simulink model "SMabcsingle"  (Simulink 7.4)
settings: Solver=ode45  StartTime=0.0  StopTime=16  MaxStep=2e-4
InitFcn:
  | smparamsingle
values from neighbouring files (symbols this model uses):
  Bm = 0.10    (= 0.1)    [IMabc2.m]    (also in imabcparam.m = 0.01; IMabcrun0.m = 0.01; IMabcrun1.m = 0.001; IMcur0.m = 1e-06)
  D = str2num(get(h,'string'))    [acttrcalc1.m]
  J = 0.02    [imabcparam.m]    (also in IMabcrun0.m; IMabcrun1.m; imdefSIvec1.m = 0.03)
  Lm = eval(get(hLm,'String'))    [im3d.m]    (also in IMabc2.m = 4.5; imabcparam.m = 0.0847; IMabcrun0.m = 0.0847; IMabcrun1.m = 0.0847)
  Lr = Lrl+Lm    (= 4.6)    [IMabc2.m]    (also in IMabcf0.m = Lrl+Lm1; IMabcf1.m = Lrl+Lm1; imabcparam.m = 0.0589666666667; IMcur0.m)
  Ls = Lsl+Lm    (= 4.6)    [IMabc2.m]    (also in IMabcf0.m = Lsl+Lm1; IMabcf1.m = Lsl+Lm1; imabcparam.m = 0.0589666666667; IMcur0.m)
  nsync = 120*freq0/p    (= 1800)    [imabcparam.m]
  p = cos(beta-alpha)    [abcRwdg.m]    (also in alternator.m = 0:pi/20:2*pi; altwdgs.m = 0:pi/20:2*pi; brushlessdcB.m = 0:pi/100:2*pi; brushlessdcnew.m = 0:pi/100:2*pi)
  R = str2num(get(h,'string'))    [acttrcalc1.m]    (also in IMabc2.m = diag([Rs Rs Rs Rr Rr Rr]); IMabcf0.m = diag([Rs Rs Rs Rr Rr Rr]); IMabcf1.m = diag([Rs Rs Rs Rr Rr Rr]); IMcurf0.m = diag([Rs Rs Rr Rr]))
  Vm = Vll*sqrt(2/3)    [imabcparam.m]
  wo = 2*pi*freq0    [calc0.m]    (also in IMabc2.m = 376.991118431; imabcparam.m = 376.991118431; IMabcrun0.m = 376.991118431; IMabcrun1.m = 376.991118431)
undefined symbols (not defined in the file or in its folder): Row, TL, vector, vr1, vr2, vr3

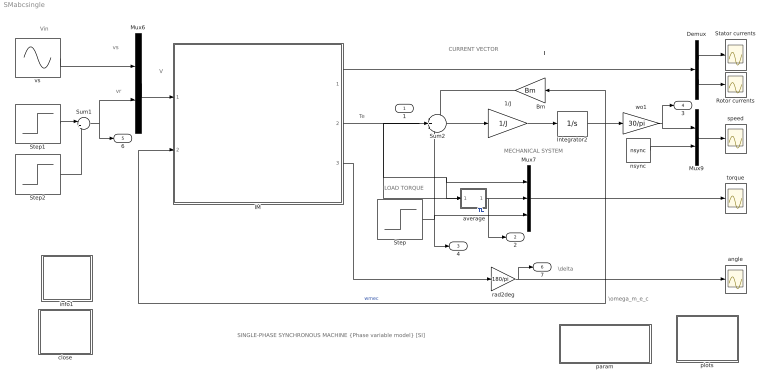
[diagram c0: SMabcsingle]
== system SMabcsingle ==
  note: SINGLE-PHASE SYNCHRONOUS MACHINE {Phase variable model} [SI]
  note: I
  note: CURRENT VECTOR
  note: V
  note: vs
  note: Vin
  note: vr
  note: Te
  note: MECHANICAL SYSTEM
  note: \omega_m_e_c
  note: LOAD TORQUE
  note: \delta
  " average" : Subsystem
  1/J : Gain  Gain=1/J  ParameterDataType=sfix(16)  ParameterScaling=2^0  OutDataType=sfix(16)  OutScaling=2^0
  Bm : Gain  Gain=Bm  ParameterDataType=sfix(16)  ParameterScaling=2^0  OutDataType=sfix(16)  OutScaling=2^0
  Demux : Demux  Outputs=2
  IM : Subsystem
  Integrator2 : Integrator  InitialCondition=wo*2/p
  Mux6 : Mux  Inputs=2
  Mux7 : Mux  Inputs=3
  Mux9 : Mux  Inputs=2
  Rotor currents : Scope
  Stator currents : Scope
  Step : Step  Time=12  After=TL  SampleTime=0
  Step1 : Step  Time=4  Before=vr1  After=vr2  SampleTime=0
  Step2 : Step  Time=8  After=vr3  SampleTime=0
  Sum1 : Sum  Inputs=|++  OutDataType=sfix(16)  OutScaling=2^0
  Sum2 : Sum  Inputs=-+-  OutDataType=sfix(16)  OutScaling=2^0
  angle : Scope
  close : Subsystem
  info1 : Subsystem
  nsync : Constant  Value=nsync  OutDataType=sfix(16)  OutScaling=2^0
  param : Subsystem
  plots : Subsystem
  rad2deg : Gain  Gain=180/pi  ParameterDataType=sfix(16)  ParameterScaling=2^0  OutDataType=sfix(16)  OutScaling=2^0
  speed : Scope
  torque : Scope
  vs : Sin  Amplitude=Vm  Bias=0  Frequency=wo  Phase=pi/2  Samples=10  SampleTime=0
  wo1 : Gain  Gain=30/pi  ParameterDataType=sfix(16)  ParameterScaling=2^0  OutDataType=sfix(16)  OutScaling=2^0
  1 : Outport
  2 : Outport  Port=2
  4 : Outport  Port=3
  3 : Outport  Port=4
  6 : Outport  Port=5
  7 : Outport  Port=6
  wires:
  Demux/1 -> Stator currents/1
  Demux/2 -> Rotor currents/1
  IM/1(I) -> Demux/1
  Mux6/1 -> IM/1(V)
  vs/1 -> Mux6/1
  Sum2/1 -> 1/J/1
  1/J/1 -> Integrator2/1
  Integrator2/1 -> wo1/1, Bm/1, IM/2(wmec)  "wmec"
  Bm/1 -> Sum2/1
  Mux9/1 -> speed/1
  wo1/1 -> 3/1, Mux9/1
  nsync/1 -> Mux9/2
  Mux7/1 -> torque/1
  " average"/1(ave) -> Mux7/2, 2/1
  Step1/1 -> Sum1/1
  Step2/1 -> Sum1/2
  Sum1/1 -> Mux6/2, 6/1
  IM/2(Te) -> Sum2/2, 1/1, Mux7/1, " average"/1(sig)
  Step/1 -> Sum2/3, Mux7/3, 4/1  "TL"
  rad2deg/1 -> angle/1, 7/1
  IM/3(delta) -> rad2deg/1

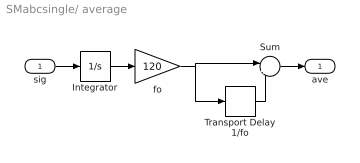
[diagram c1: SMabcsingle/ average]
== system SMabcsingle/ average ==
  sig : Inport  OutDataType=sfix(16)  OutScaling=2^0
  Integrator : Integrator
  Sum : Sum  Inputs=|+-  OutDataType=sfix(16)  OutScaling=2^0
  Transport Delay 1/fo : TransportDelay  DelayTime=1/120
  fo : Gain  Gain=120  ParameterDataType=sfix(16)  ParameterScaling=2^0  OutDataType=sfix(16)  OutScaling=2^0
  ave : Outport
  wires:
  Sum/1 -> ave/1
  Transport Delay 1/fo/1 -> Sum/2
  sig/1 -> Integrator/1
  fo/1 -> Transport Delay 1/fo/1, Sum/1
  Integrator/1 -> fo/1

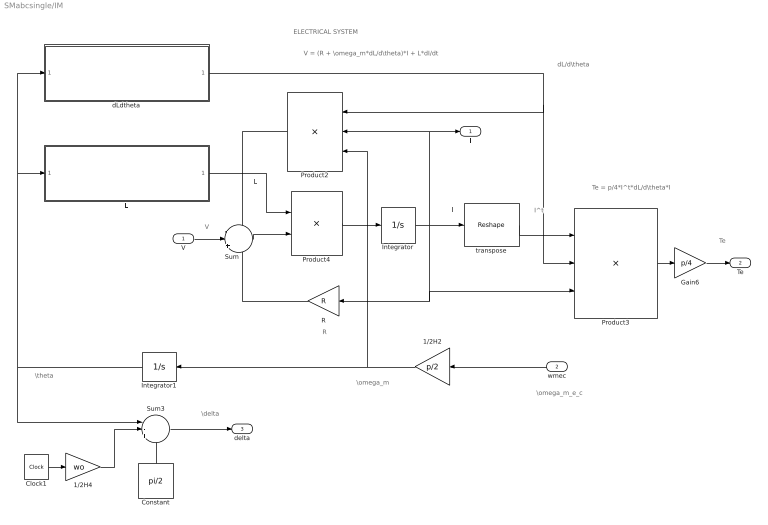
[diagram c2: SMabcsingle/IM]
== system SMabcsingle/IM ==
  note: I
  note: I^t
  note: ELECTRICAL SYSTEM
  note: V
  note: \theta
  note: L
  note: Te
  note: R
  note: V = (R + \omega_m*dL/d\theta)*I + L*dI/dt
  note: Te = p/4*I^t*dL/d\theta*I
  note: \omega_m_e_c
  note: dL/d\theta
  note: \omega_m
  note: \delta
  V : Inport  OutDataType=sfix(16)  OutScaling=2^0
  wmec : Inport  Port=2  OutDataType=sfix(16)  OutScaling=2^0
  1/2H2 : Gain  Gain=p/2  ParameterDataType=sfix(16)  ParameterScaling=2^0  OutDataType=sfix(16)  OutScaling=2^0
  1/2H4 : Gain  Gain=wo  ParameterDataType=sfix(16)  ParameterScaling=2^0  OutDataType=sfix(16)  OutScaling=2^0
  Clock1 : Clock
  Constant : Constant  Value=pi/2  OutDataType=sfix(16)  OutScaling=2^0
  Gain6 : Gain  Gain=p/4  ParameterDataType=sfix(16)  ParameterScaling=2^0  OutDataType=sfix(16)  OutScaling=2^0
  Integrator : Integrator  InitialCondition=[0 ;0 ]
  Integrator1 : Integrator  InitialCondition=-pi/2
  L : Subsystem
  Product2 : Product  Inputs=***  Multiplication=Matrix(*)  OutDataType=sfix(16)  OutScaling=2^0
  Product3 : Product  Inputs=3  Multiplication=Matrix(*)  OutDataType=sfix(16)  OutScaling=2^0
  Product4 : Product  Inputs=/*  Multiplication=Matrix(*)  OutDataType=sfix(16)  OutScaling=2^0
  R : Gain  Gain=R  Multiplication=Matrix(K*u)  ParameterDataType=sfix(16)  ParameterScaling=2^0  OutDataType=sfix(16)  OutScaling=2^0
  Sum : Sum  Inputs=-|+|-  OutDataType=sfix(16)  OutScaling=2^0
  Sum3 : Sum  Inputs=|-+-  OutDataType=sfix(16)  OutScaling=2^0
  dLdtheta : Subsystem
  transpose : Reshape  OutputDimensionality=Row vector (2-D)  OutputDimensions=[1,6]
  I : Outport
  Te : Outport  Port=2
  delta : Outport  Port=3
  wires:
  Product4/1 -> Integrator/1
  Integrator/1 -> Product3/3, R/1, Product2/2, I/1, transpose/1
  Sum/1 -> Product4/2
  R/1 -> Sum/3
  transpose/1 -> Product3/1
  Product2/1 -> Sum/1
  dLdtheta/1(dLdtheta) -> Product3/2, Product2/1
  Product3/1 -> Gain6/1
  Integrator1/1 -> dLdtheta/1(theta1), L/1(theta), Sum3/1
  L/1(L) -> Product4/1
  V/1 -> Sum/2
  Gain6/1 -> Te/1
  wmec/1 -> 1/2H2/1
  1/2H2/1 -> Integrator1/1, Product2/3
  Clock1/1 -> 1/2H4/1
  1/2H4/1 -> Sum3/2
  Constant/1 -> Sum3/3
  Sum3/1 -> delta/1

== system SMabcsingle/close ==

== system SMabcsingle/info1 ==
  note: This demo simulates the operation of an elementary single-phase synchronous machine. It consists of a single stator winding of self inductance Ls and a single rotor winding of inductance Lr. The mutual coupling between the two windings is given as Lm*cos(theta) where theta is the angle between the axes of the windings. Saliency and saturation are thus ignored. The stator winding is connected to a sinusoidal voltage source vs=Vm*cos(wo.t) and the rotor winding to a dc voltage vr. The machine operates as a motor connected to a mechanical load, and runs at synchronous speed. The specific operation examined here consists of having the motor run first at no load (TL=0) and establishing with vr 3 excitation levels in succession: under excitation vr vro (is leads vs). A mechanical load is then suddenly applied as a step (TL=1.6 N.m). Because of the absence of damping elements, the average torque developed is oscillatory. Estimate the period of these oscillations and verify that the frequency of the stator current is wo , the rotor current 2*wo, and the instatntaneous torque 2*wo . Other configurations and operating conditions of this machine can be further examined. Note that dq analysis is not applicable to this most elementary system.

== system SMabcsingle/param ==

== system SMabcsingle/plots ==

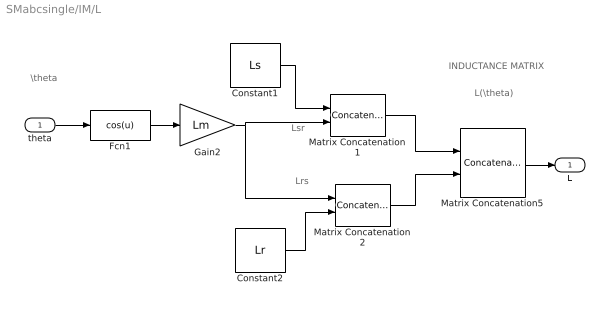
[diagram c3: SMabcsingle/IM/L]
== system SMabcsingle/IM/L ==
  note: INDUCTANCE MATRIX
  note: Lsr
  note: Lrs
  note: \theta
  note: L(\theta)
  theta : Inport  OutDataType=sfix(16)  OutScaling=2^0
  Constant1 : Constant  Value=Ls  VectorParams1D=off  OutDataType=sfix(16)  OutScaling=2^0
  Constant2 : Constant  Value=Lr  VectorParams1D=off  OutDataType=sfix(16)  OutScaling=2^0
  Fcn1 : Fcn  Expr=cos(u)
  Gain2 : Gain  Gain=Lm  ParameterDataType=sfix(16)  ParameterScaling=2^0  OutDataType=sfix(16)  OutScaling=2^0
  Matrix Concatenation1 : Concatenate  Mode=Multidimensional array  ConcatenateDimension=2
  Matrix Concatenation2 : Concatenate  Mode=Multidimensional array  ConcatenateDimension=2
  Matrix Concatenation5 : Concatenate  Mode=Multidimensional array
  L : Outport
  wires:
  Matrix Concatenation5/1 -> L/1
  Gain2/1 -> Matrix Concatenation1/2, Matrix Concatenation2/1
  Matrix Concatenation1/1 -> Matrix Concatenation5/1
  Matrix Concatenation2/1 -> Matrix Concatenation5/2
  Constant1/1 -> Matrix Concatenation1/1
  Constant2/1 -> Matrix Concatenation2/2
  theta/1 -> Fcn1/1
  Fcn1/1 -> Gain2/1

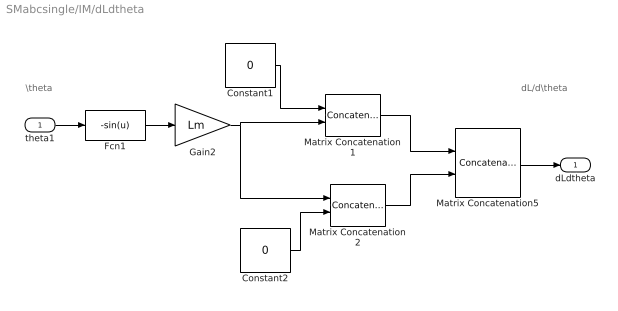
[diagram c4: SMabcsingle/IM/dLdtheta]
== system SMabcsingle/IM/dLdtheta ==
  note: dL/d\theta
  note: \theta
  theta1 : Inport  OutDataType=sfix(16)  OutScaling=2^0
  Constant1 : Constant  Value=0  VectorParams1D=off  OutDataType=sfix(16)  OutScaling=2^0
  Constant2 : Constant  Value=0  VectorParams1D=off  OutDataType=sfix(16)  OutScaling=2^0
  Fcn1 : Fcn  Expr=-sin(u)
  Gain2 : Gain  Gain=Lm  ParameterDataType=sfix(16)  ParameterScaling=2^0  OutDataType=sfix(16)  OutScaling=2^0
  Matrix Concatenation1 : Concatenate  Mode=Multidimensional array  ConcatenateDimension=2
  Matrix Concatenation2 : Concatenate  Mode=Multidimensional array  ConcatenateDimension=2
  Matrix Concatenation5 : Concatenate  Mode=Multidimensional array
  dLdtheta : Outport
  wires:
  Gain2/1 -> Matrix Concatenation1/2, Matrix Concatenation2/1
  Matrix Concatenation1/1 -> Matrix Concatenation5/1
  Matrix Concatenation2/1 -> Matrix Concatenation5/2
  Constant1/1 -> Matrix Concatenation1/1
  Constant2/1 -> Matrix Concatenation2/2
  Fcn1/1 -> Gain2/1
  theta1/1 -> Fcn1/1
  Matrix Concatenation5/1 -> dLdtheta/1
